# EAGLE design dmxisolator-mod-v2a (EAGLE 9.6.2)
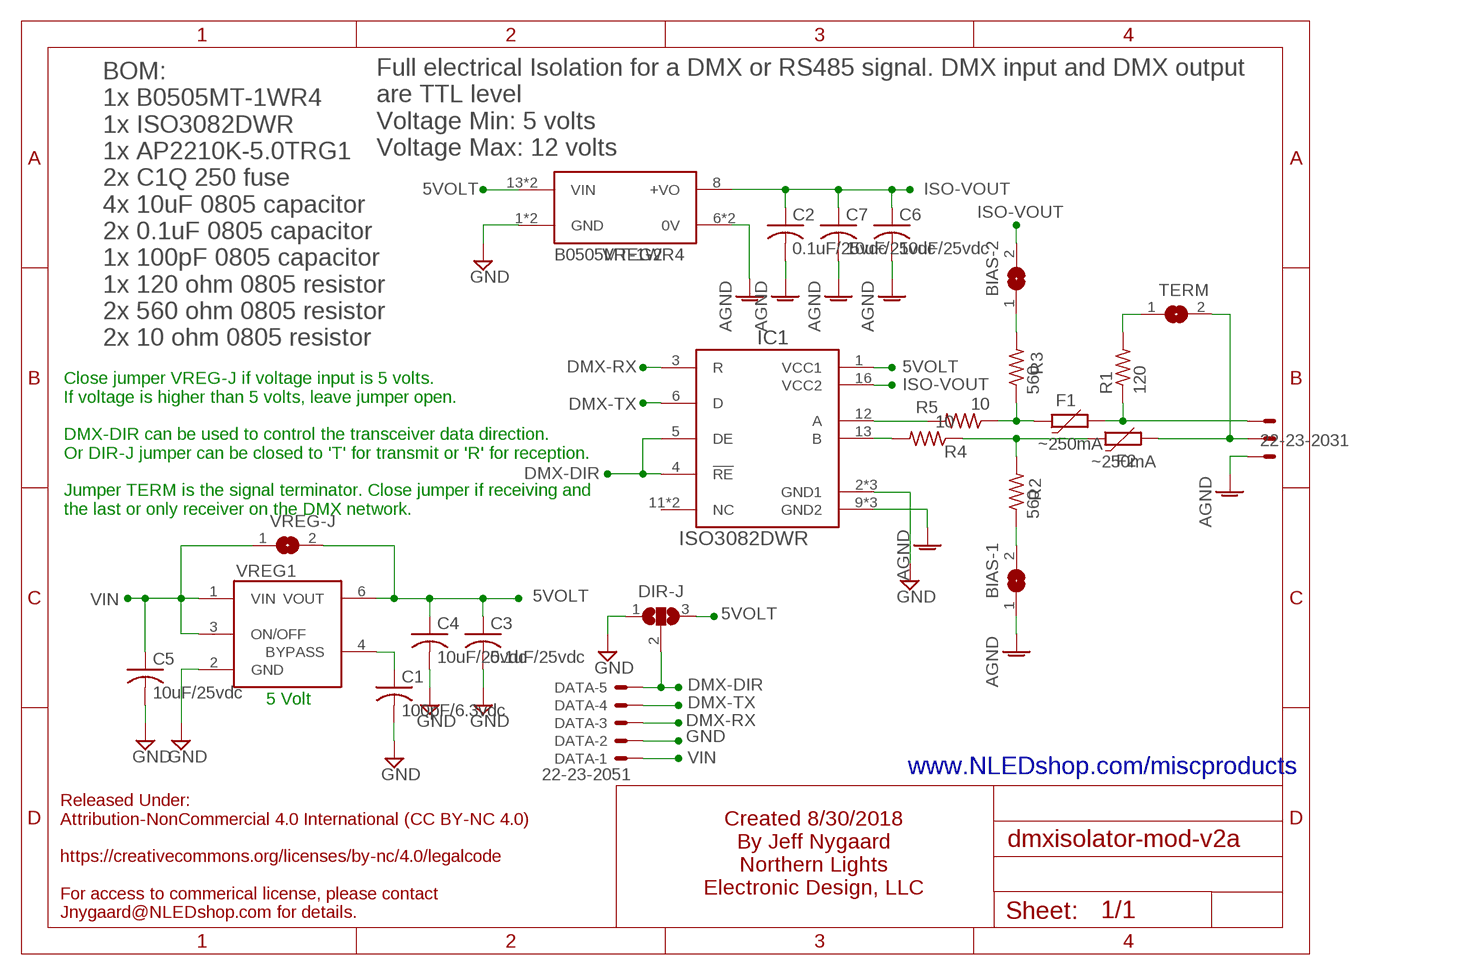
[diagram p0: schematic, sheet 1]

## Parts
BIAS-1  SMD-JUMPER-NOPASTEINSET2  [SJ-INSET-2-NOPASTE]
BIAS-2  SMD-JUMPER-NOPASTEINSET2  [SJ-INSET-2-NOPASTE]
C1  100pF/6.3vdc  C-USC0805  [C0805]
C2  0.1uF/25vdc  C-USC0805  [C0805]
C3  0.1uF/25vdc  C-USC0805  [C0805]
C4  10uF/25vdc  C-USC0805  [C0805]
C5  10uF/25vdc  C-USC0805  [C0805]
C6  10uF/25vdc  C-USC0805  [C0805]
C7  10uF/25vdc  C-USC0805  [C0805]
DATA  22-23-2051  [22-23-2051]
DIR-J  SJ2W  [SJ_2]
DMX  22-23-2031  [22-23-2031]
F1  ~250mA  PTC-FUSE  [R1206]
F2  ~250mA  PTC-FUSE  [R1206]
IC1  ISO3082DWR  [SOIC127P1030X265-16N]
R1  120  R-US_R0805  [R0805]
R2  560  R-US_R0805  [R0805]
R3  560  R-US_R0805  [R0805]
R4  10  R-US_R0805  [R0805]
R5  10  R-US_R0805  [R0805]
TERM  SMD-JUMPER-NOPASTEINSET2  [SJ-INSET-2-NOPASTE]
VREG1  AP2210K  [SOT-23-5]
VREG2  B0505MT-1WR4  [CONV_B0505MT-1WR4]
VREG-J  SMD-JUMPER-NOPASTE  [SJ-NOPASTE]

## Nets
5VOLT: C3.1 C4.1 DIR-J.3 IC1.1(VCC1) VREG1.6(VOUT) VREG2.13(VIN) VREG2.14(VIN) VREG-J.2
AGND: BIAS-1.1 C2.2 C6.2 C7.2 DMX.1 IC1.9(GND2) IC1.10(GND2) IC1.15(GND2) VREG2.6(0V) VREG2.7(0V)
BYPASS: C1.1 VREG1.4(BYPASS)
DMX-DIR: DATA.5 DIR-J.2 IC1.4(!RE) IC1.5(DE)
DMX-INV: DMX.3 F2.2 TERM.2
DMX-POS: DMX.2 F1.2 R1.1
DMX-RX: DATA.3 IC1.3(R)
DMX-TX: DATA.4 IC1.6(D)
GND [ground]: C1.2 C3.2 C4.2 C5.2 DATA.2 DIR-J.1 IC1.2(GND1) IC1.7(GND1) IC1.8(GND1) VREG1.2(GND) VREG2.1(GND) VREG2.2(GND)
ISO-VOUT: BIAS-2.2 C2.1 C6.1 C7.1 IC1.16(VCC2) VREG2.8(+VO)
N$1: R1.2 TERM.1
N$2: BIAS-1.2 R2.1
N$3: IC1.13(B) R4.2
N$4: IC1.12(A) R5.2
N$5: BIAS-2.1 R3.2
N$6: F1.1 R3.1 R5.1
N$7: F2.1 R2.2 R4.1
VIN: C5.1 DATA.1 VREG1.1(VIN) VREG1.3(ON/OFF) VREG-J.1
Unconnected: IC1.11(NC) IC1.14(NC)

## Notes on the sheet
- Full electrical Isolation for a DMX or RS485 signal. DMX input and DMX output
  are TTL level
  Voltage Min: 5 volts
  Voltage Max: 12 volts
- BOM:
  1x B0505MT-1WR4
  1x ISO3082DWR  
  1x AP2210K-5.0TRG1 
  2x C1Q 250 fuse
  4x 10uF 0805 capacitor
  2x 0.1uF 0805 capacitor
  1x 100pF 0805 capacitor
  1x 120 ohm 0805 resistor
  2x 560 ohm 0805 resistor
  2x 10 ohm 0805 resistor
- Close jumper VREG-J if voltage input is 5 volts.
  If voltage is higher than 5 volts, leave jumper open.
  
  DMX-DIR can be used to control the transceiver data direction.
  Or DIR-J jumper can be closed to 'T' for transmit or 'R' for reception.
  
  Jumper TERM is the signal terminator. Close jumper if receiving and
  the last or only receiver on the DMX network.
- 5 Volt
- www.NLEDshop.com/miscproducts
- Created 8/30/2018
  By Jeff Nygaard
  Northern Lights
  Electronic Design, LLC
- Released Under:
  Attribution-NonCommercial 4.0 International (CC BY-NC 4.0)
  
  https://creativecommons.org/licenses/by-nc/4.0/legalcode
  
  For access to commerical license, please contact
  Jnygaard@NLEDshop.com for details.

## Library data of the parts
BIAS-1 BIAS-2 TERM VREG-J = NLED-connectors:SMD-JUMPER-NOPASTE: SMD solder JUMPER
C1-C7 = rcl:C-US: CAPACITOR, American symbol; SPICEPREFIX: C
DATA = con-molex:22-23-2051: .100" (2.54mm) Center Header - 5 Pin; MF: MOLEX; MPN: 22-23-2051; OC_FARNELL: 1462952; OC_NEWARK: 38C9178
DIR-J = jumper:SJ2W: SMD solder JUMPER
DMX = con-molex:22-23-2031: .100" (2.54mm) Center Header - 3 Pin; MF: MOLEX; MPN: 22-23-2031; OC_FARNELL: 1462950; OC_NEWARK: 30C0862
F1 F2 = NLED-inductors-ferrites-diodes:PTC-FUSE
IC1 = ISO3082DWR:ISO3082DWR; MANUFACTURER: Texas Instruments; MAXIMUM_PACKAGE_HEIGHT: 2.65 mm; PARTREV: I; STANDARD: Manufacturer Recommendations
R1-R5 = rcl:R-US_: RESISTOR, American symbol; SPICEPREFIX: R
VREG1 = NLED-integratedcircuit:AP2210K: AP2210K - Diodes Incorporated LDO Voltage Regulators 300mA CMOS LDO 5.0V 250mV
VREG2 = B0505MT-1WR4:B0505MT-1WR4: DC/DC Converter; MANUFACTURER: Mornsun; MAXIMUM_PACKAGE_HEIGHT: 3.40 mm; PARTREV: 2020.10.10-A/2; STANDARD: Manufacturer Recommendations

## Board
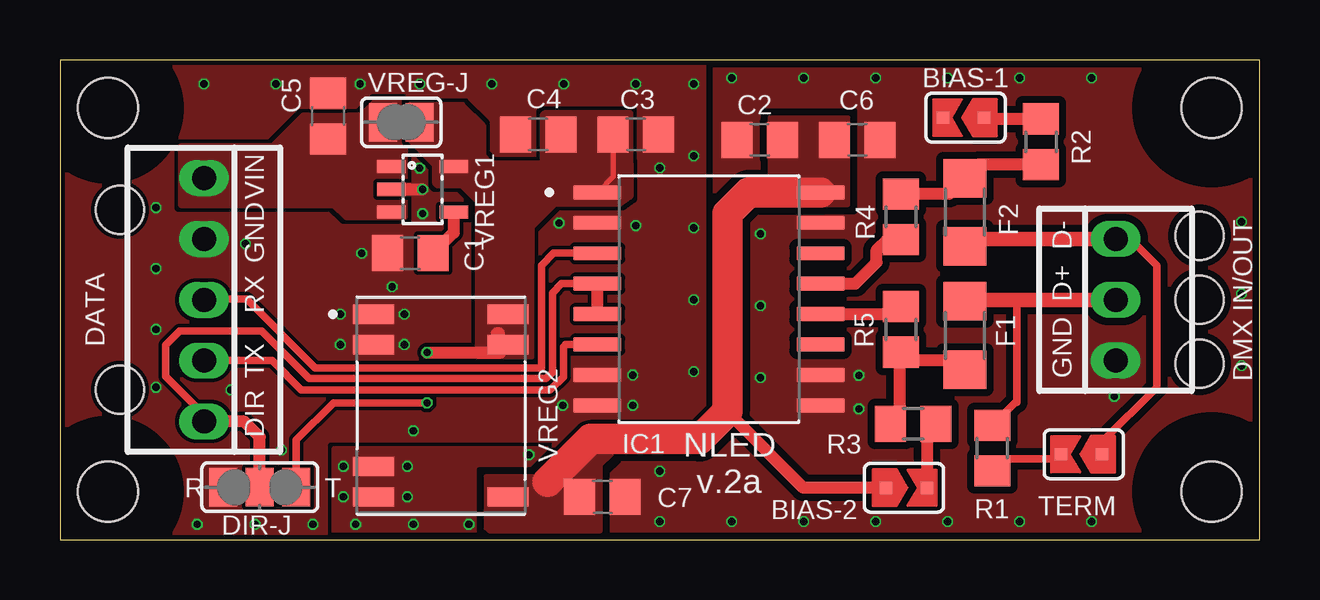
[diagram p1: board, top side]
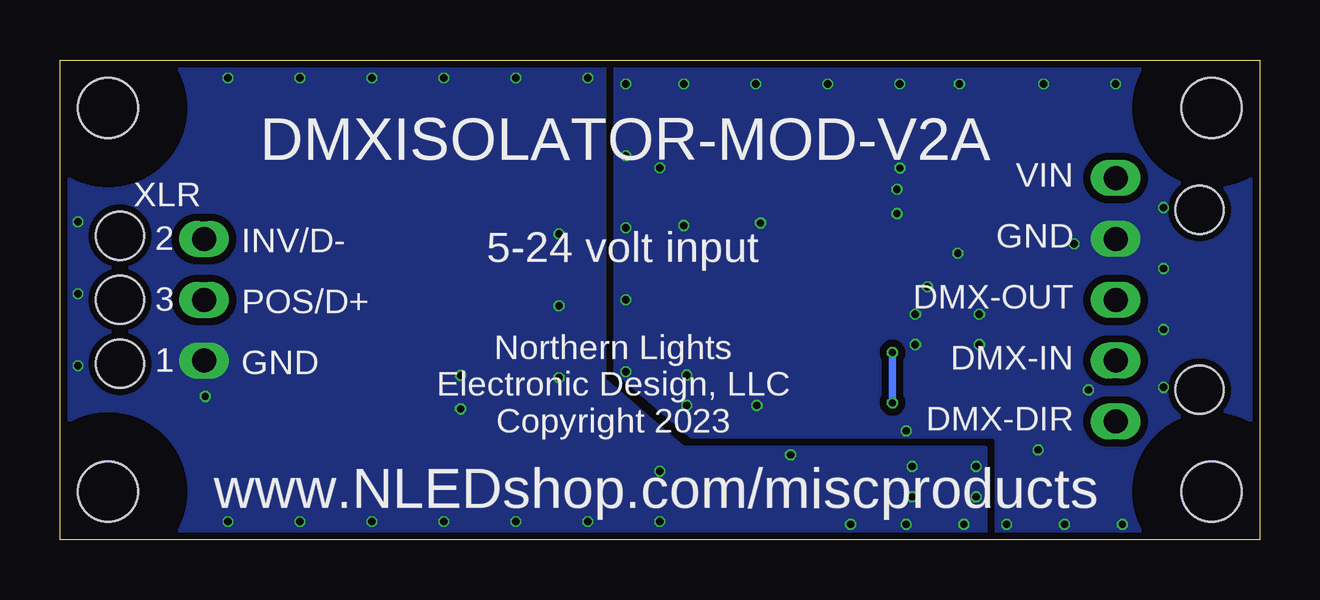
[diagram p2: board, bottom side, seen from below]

Size 50 x 20 mm. Coordinates in mm from the lower left corner, seen from the top.
Outline: 0,0 50,0 50,20 0,20 0,0
Copper layers (1*16): Top 0.035mm / dielectric 1.6mm / Bottom 0.035mm
Design rules "nled-2layer": minimum track width 6mil, minimum drill 0.3mm, track to track 6mil, track to pad 6mil, pad to pad 6mil, via to via 6mil, smd to smd 6mil, copper to edge 0.2mm, drill to drill 6mil, minimum pad ring 10mil, minimum via ring 3mil, stop-mask expansion 4mil, vias tented up to drill 100mil, thermal gap 10mil
Holes 2 mm at 2.5,6.25 2.5,13.75 47.5,12.67 47.5,10 47.5,7.33
Holes 2.5 mm at 48,2 2,18 2,2 48,18
tRestrict: area -1,-1 to 5,5; area -1,15 to 5,21; area 45,15 to 51,21; area 45,-1 to 51,5
bRestrict: area 45,-1 to 51,5; area 45,15 to 51,21; area -1,15 to 5,21; area -1,-1 to 5,5

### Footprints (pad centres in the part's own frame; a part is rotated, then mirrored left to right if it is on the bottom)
SJ-INSET-2-NOPASTE = smd 0.5 x 0.5: 1 -0.95,0; 2 0.762,0
C0805 = smd 1.3 x 1.5: 1 -0.95,0; 2 0.95,0
22-23-2051 = drill 1 long: 1 -5.08,0; 2 -2.54,0; 3 0,0; 4 2.54,0; 5 5.08,0
SJ_2 = smd 1.168 x 1.6: 1 -1.524,0; 2 0,0; 3 1.524,0
22-23-2031 = drill 1 long: 1 -2.54,0; 2 0,0; 3 2.54,0
R1206 = smd 1.6 x 1.803: 1 -1.422,0; 2 1.422,0
SOIC127P1030X265-16N = smd 2 x 0.6: 1 -4.65,4.445; 2 -4.65,3.175; 3 -4.65,1.905; 4 -4.65,0.635; 5 -4.65,-0.635; 6 -4.65,-1.905; 7 -4.65,-3.175; 8 -4.65,-4.445; 9 4.65,-4.445; 10 4.65,-3.175; 11 4.65,-1.905; 12 4.65,-0.635; 13 4.65,0.635; 14 4.65,1.905; 15 4.65,3.175; 16 4.65,4.445
R0805 = smd 1.3 x 1.5: 1 -0.95,0; 2 0.95,0
SOT-23-5 = smd 0.55 x 1.2: 1 -0.95,-1.3; 2 0,-1.3; 3 0.95,-1.3; 4 0.95,1.3; 6 -0.95,1.3
CONV_B0505MT-1WR4 = smd 1.7 x 0.8: 1 -2.8,3.81; 2 -2.8,2.54; 6 -2.8,-2.54; 7 -2.8,-3.81; 8 2.8,-3.81; 13 2.8,2.54; 14 2.8,3.81
SJ-NOPASTE = smd 1.168 x 1.6: 1 -0.762,0; 2 0.762,0

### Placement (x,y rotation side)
BIAS-1  37.75,17.59 0 top
BIAS-2  35.18,2.16 180 top
C1  14.61,11.94 180 top
C2  29.16,16.66 180 top
C3  24,16.89 0 top
C4  19.94,16.89 180 top
C5  11.18,17.65 90 top
C6  33.23,16.66 0 top
C7  22.61,1.78 0 top
DATA  6,10 270 top
DIR-J  8.33,2.19 0 top
DMX  44,10 90 top
F1  37.72,8.51 90 top
F2  37.72,13.64 270 top
IC1  27.05,10.03 0 top
R1  38.86,3.81 270 top
R2  40.89,16.59 270 top
R3  35.56,4.83 0 top
R4  35.05,13.46 270 top
R5  35.05,8.76 90 top
TERM  42.67,3.56 0 top
VREG1  15.11,14.61 270 top
VREG2  15.88,5.59 0 top
VREG-J  14.22,17.4 0 top

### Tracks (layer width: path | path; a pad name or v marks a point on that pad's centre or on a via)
5VOLT  (via drill 0.3)
  Top 0.203: C3.1 23.05,15.13 IC1.1
  Top 0.305: v15.3,5.7 11.4,5.7 9.85,4.15 DIR-J.3
  Top 0.508: 18.2,8.6 18.3,8.6 | v15.3,7.8 18.35,7.8 VREG2.13
  Bottom 0.305: v15.3,5.7 v15.3,7.8
  pour Top (no thermals): 17.4,7.62 17.4,14.1 16.76,14.73 15.75,14.73 15.62,14.86 15.62,15.62 14.61,16.64 14.61,18.16 16.76,18.16 17.65,17.27 17.65,16 17.91,15.75 23.8,15.7 23.8,14.3 23.34,13.97 20.62,13.97 19.68,13.04 19.68,7.62
  pour Top (no thermals): 20.1,17.7 20.1,15.8 23.8,15.8 23.8,17.8 20.2,17.8
AGND  (via drill 0.3)
  other vias: 11.81,3.05 11.81,1.78 14.48,1.78 14.48,3.05 12.32,0.64 14.73,0.64 17.05,0.64 25,0.75 28,0.75 31,0.75 34,0.75 37,0.75 40,0.75 43,0.75 43.94,5.97 28,19.25 31,19.25 34,19.25 37,19.25 40,19.25 43,19.25 49.25,13.25 49.25,10.25 49.25,7.25 29.2,12.75 29.2,9.75 29.2,6.75 33.3,6.85 33.3,5.45 25,2.85 19.55,3.54
  pour Bottom (isolate 0.3, rank 2, no thermals): 50,0 11.43,0 11.43,3.81 24.04,3.81 27.32,6.64 27.32,20 50,20
  pour Top (isolate 0.3, rank 2, no thermals): 50,0 11.43,0 11.43,3.81 25.4,3.81 27.32,5.46 27.32,15.89 27.32,20 50,20
BYPASS
  Top 0.508: VREG1.4 16.41,12.8 C1.1
DMX-DIR
  Top 0.305: IC1.4 20.9,10.67 20.52,10.29 20.52,6.98 20.25,6.71 10.39,6.71 8.4,8.7 4.99,8.7 4.4,8.12 4.4,6.8 6,5.2 DATA.5
  Top 0.508: IC1.5 IC1.4 | DIR-J.2 8.33,4.27 7.68,4.92 DATA.5
DMX-INV
  Top 0.305: TERM.2 43.43,4.06 45.72,6.35 45.72,11.43 44.61,12.54 43.18,12.54
  Top 0.61: F2.2 38.04,12.54 43.18,12.54 DMX.3
DMX-POS
  Top 0.305: R1.1 39.85,5.75 39.88,5.71 39.88,10
  Top 0.61: DMX.2 39.88,10 37.79,10 F1.2
DMX-RX
  Top 0.305: IC1.3 20.57,11.94 20.07,11.43 20.07,7.17 10.64,7.17 7.77,10.03 6.03,10.03 DATA.3
DMX-TX
  Top 0.305: IC1.6 21.08,8.13 20.98,8.03 20.98,6.79 20.44,6.24 10.06,6.24 8.84,7.46 DATA.4
GND  (via drill 0.3)
  Top 0.508: VREG1.2 v15.11,14.61
  other vias: 14.99,15.49 13.84,10.54 12.57,11.94 11.68,8.13 14.35,8.13 14.35,9.4 11.68,9.4 23.88,5.59 23.88,6.86 20.95,5.59 4,6.35 4,8.76 4,11.3 4,13.84 6,19 9,19 12.51,19 15,19 18,19 21,19 24,19 26.42,19 15.11,13.59 5.71,0.64 8.13,0.64 10.54,0.64 20.8,13.2 24,13.1 25,15.5 26.42,16 26.42,13 26.42,10 26.42,7 9.23,3.73 7.13,6.24 14.73,4.54 7.73,12.34
  pour Bottom (isolate 0.3, rank 6, no thermals): 0,20.07 0,0 26.84,0 26.84,20.07
  pour Top (isolate 0.15, rank 6, no thermals): 0,20.07 0,0 26.84,0 26.84,20.07
ISO-VOUT
  Top 0.508: BIAS-2.2 30.99,2.16 27.81,5.33
  Top 1.27: IC1.16 28.7,14.48 27.81,13.59 27.81,5.33 26.67,4.19 22.11,4.19 20.32,2.4
  pour Top (no thermals): 17.78,2.6 17.78,0.51 17.91,0.38 22.5,0.38 22.5,3.1 23,3.6 21.8,3.6 20.8,2.6
  pour Top (no thermals): 29.59,17.58 29.59,13.97 32.85,13.97 32.85,17.58
N$1
  Top 0.305: TERM.1 41.52,3.36 39.41,3.36 38.91,2.86 R1.2
N$2
  Top 0.508: R2.1 38.56,17.54 BIAS-1.2
N$3
  Top 0.508: IC1.13 33.15,10.67 34.04,11.56 34.04,12.06 34.48,12.51 R4.2
N$4
  Top 0.508: IC1.12 34.74,9.4 R5.2
N$5
  Top 0.508: R3.2 36.13,4.45 BIAS-2.1
N$6
  Top 0.508: R3.1 34.99,5.21 34.99,7.55 35.05,7.49 | 35.05,7.49 R5.1 | F1.1 37.34,7.47 35.08,7.47 35.05,7.49
N$7
  Top 0.508: R4.1 37.07,14.41 F2.1 38.29,15.64 R2.2
VIN
  pour Top (rank 5, no thermals): 5.08,16.38 5.08,13.97 11.43,13.97 11.94,13.46 14.35,13.46 14.35,18.29 13.21,18.29 12.57,17.65 10.16,17.65 8.89,16.38

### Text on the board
tPlace: DMX IN/OUT | NLED / v.2a
tNames: VIN | GND | RX | TX | GND D+ D- | DIR | R | T
bNames: DMXISOLATOR-MOD-V2A | XLR | 5-24 volt input | INV/D- / POS/D+ / GND | 2 / 3 / 1 | Northern Lights / Electronic Design, LLC / Copyright 2023 | VIN / GND / DMX-OUT / DMX-IN / DMX-DIR | www.NLEDshop.com/miscproducts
